(* Logix 5000 DataType export CIP_Axis; software revision 34.01 *)

TYPE CIP_Axis :   // CIP Sync Axis Object
STRUCT
   Control : CIP_Control;   // Control bits to send to the drive
   Status : CIP_Status;   // Status bits received from the drive
   Input : CIP_AxisInputData;   // Data from the drive
   Output : CIP_AxisOutputData;   // Data to the drive
   PositionFeedback : DINT;   // Actual Position Value
   PositionCommand : DINT;   // Drive's commanded position
   ResponseTimestamp : LINT;   // Drive's timestamp of response
   RequestedAction : INT;   // State_Machine_Requested_Action
END_STRUCT
END_TYPE

TYPE CIP_AxisInputData :
STRUCT
   Data : SINT[10];
END_STRUCT
END_TYPE

TYPE CIP_AxisOutputData :
STRUCT
   Data : SINT[14];
END_STRUCT
END_TYPE

TYPE CIP_Control :
STRUCT
   Switch_On : BOOL;
   Disable_Voltage : BOOL;
   Quick_Stop : BOOL;
   Enable_Operation : BOOL;
   Op_Mode_Specific_4 : BOOL;   // Home Start or Follow Position bit, depending on on whether bit 11 (Mode Home) or bit 12 (C
   Op_Mode_Specific_5 : BOOL;   // Unused
   Op_Mode_Specific_6 : BOOL;   // Unused
   Reset_Fault : BOOL;
   Pause_Halt : BOOL;
   Op_Mode_Specific_9 : BOOL;   // Unused
   Reserved_10 : BOOL;
   Manu_Specific_11 : BOOL;   // Mode Home bit
   Manu_Specific_12 : BOOL;   // Mode Cyclic Position bit
   Manu_Specific_13 : BOOL;   // Unused
   Manu_Specific_14 : BOOL;   // Unused
   Manu_Specific_15 : BOOL;   // Unused
END_STRUCT
END_TYPE

TYPE CIP_DynamicMap :
STRUCT
   Input : CIP_MapInputData;   // Map data from the drive
   Output : CIP_MapOutputData;   // Map data to the drive
END_STRUCT
END_TYPE

TYPE CIP_MapInputData :   // Map data received from the drive
STRUCT
   Data : SINT[40];
END_STRUCT
END_TYPE

TYPE CIP_MapOutputData :   // Map data going to drive
STRUCT
   Data : SINT[32];
END_STRUCT
END_TYPE

TYPE CIP_Status :   // All connections to the drive ethernet module are established and data is successfully transferring.
STRUCT
   Ready_To_Switch_On : BOOL;
   Switched_On : BOOL;
   Operation_Enabled : BOOL;
   Fault : BOOL;
   Voltage_Enabled : BOOL;
   Quick_Stop : BOOL;
   Switch_On_Disabled : BOOL;
   Warning : BOOL;
   STO_Active : BOOL;
   Remote : BOOL;
   Target_Reached : BOOL;
   Internal_Limit_Active : BOOL;
   Op_Mode_Specific_12 : BOOL;   // Home Attained bit
   Op_Mode_Specific_13 : BOOL;   // Homing/Cyclic Position Error bit
   Manu_Specific_14 : BOOL;   // Motion Mode bit (0 for Homing, 1 for Cyclic Position)
   Manu_Specific_15 : BOOL;   // Following Position bit (for Cyclic Position mode)
END_STRUCT
END_TYPE
